PROGRAM MAIN
VAR
	axis: AXIS_REF;
	fbAxisPower: MC_Power;
	fbAxisMoveAbsolute: MC_MoveAbsolute;
	bEnable: BOOL := FALSE;
	fOverride: LREAL := 100;
	bMove: BOOL := FALSE;
	fTargetPosition: LREAL := 90;
	fTargetVelocity: LREAL := 5;
	iMotorDriveSubmodeSelect AT%Q*:UDINT;

END_VAR

axis.ReadStatus();

fbAxisPower(
	Axis:= axis,
	Enable:= bEnable,
	Enable_Positive:= bEnable,
	Enable_Negative:= bEnable,
	Override:= fOverride,
	BufferMode:= ,
	Options:= ,
	Status=> ,
	Busy=> ,
	Active=> ,
	Error=> ,
	ErrorID=> 
);
	
fbAxisMoveAbsolute(
	Axis:= axis,
	Execute:= bMove,
	Position:= fTargetPosition,
	Velocity:= fTargetVelocity,
	Acceleration:= ,
	Deceleration:= ,
	Jerk:= ,
	BufferMode:= ,
	Options:= ,
	Done=> ,
	Busy=> ,
	Active=> ,
	CommandAborted=> ,
	Error=> ,
	ErrorID=> 
);

END_PROGRAM
